(* Logix 5000 AddOnInstructionDefinition export YAI_Assy_72_73_22_23_EIP_Hz; software revision 17.00 *)

ADD_ON_INSTRUCTION YAI_Assy_72_73_22_23_EIP_Hz   (* revision 1.0, vendor Yaskawa America, Inc. *)
// YAI Assembly 72/73 and 22/23
// Speed is given in Hz
// Torque is given in % rated torque
// Help:
// This add-on instruction is for use with input assemblie 72 or 73 and output assemblies 22 or 23.
// Node_Input_Assy is defined as the node's input assembly integer array.
// Node_Output_Assy is defined as the node's output assembly integer array.
// Torque limit/reference and torque output variables are only available with A1000.
VAR_IN_OUT
   Node_Input_Assy : AB:ETHERNET_MODULE_INT_6Bytes:I:0; {required}   // Input assembly words
   Node_Output_Assy : AB:ETHERNET_MODULE_INT_6Bytes:O:0; {required}   // Output assembly words
END_VAR
VAR_INPUT
   RunFwd : BOOL; {visible}   // Forward run command
   RunRev : BOOL; {visible}   // Reverse run command
   FaultReset : BOOL; {visible}   // Fault reset command
   Net_Control : BOOL;   // Network control bit to switch between b1-02 setting and network.
   Net_Ref : BOOL;   // Network reference bit to switch between b1-01 setting and network.
   Freq_Ref : REAL; {visible}   // Frequency reference command in Hz (xx.xx resolution)
   Torq_Ref_Limit : REAL; {visible}   // Torque reference/limit (A1000 only) Engineering Units
END_VAR
VAR_OUTPUT
   Faulted : BOOL; {visible}   // Drive faulted status bit
   Warning : BOOL; {visible}   // Drive warning (alarm) status bit
   RunningFwd : BOOL; {visible}   // Drive running forward status bit
   RunningRev : BOOL; {visible}   // Drive running reverse status bit
   Ready : BOOL; {visible}   // Drive ready status bit
   NetRefStatus : BOOL; {visible}   // Drive network reference status bit (1 = reference coming from network)
   NetCtrlStatus : BOOL; {visible}   // Drive network run source status bit (1 = source coming from network)
   Drive_State : INT;   // Drive Status - Refer to class 0x29, Instance 0x1, Attribute 0x6 for details
   At_Speed : BOOL; {visible}   // Drive at commanded speed status bit
   Output_Freq : REAL; {visible}   // Drive output frequency in Hz (xx.xx resolution)
   Torque_Actual : REAL; {visible}   // Drive torque output in engineering units.
END_VAR
VAR_INPUT
   Motor_Rated_Torq : REAL := 100.0; {visible}   // Motor rated torque (Engineering units)
END_VAR
VAR
   FRef_Convert : DINT;
   FOut_Convert : REAL;
   FOut_Temp : REAL;
   TRef_Convert : INT;
   DriveStatusTempBits : INT;
   TOut_Convert : REAL;
   TOut_Temp : REAL;
   Motor_Torq_Temp : REAL;
   Tout_Convert_Temp : REAL;
END_VAR

ROUTINE Logic   (* ladder *)
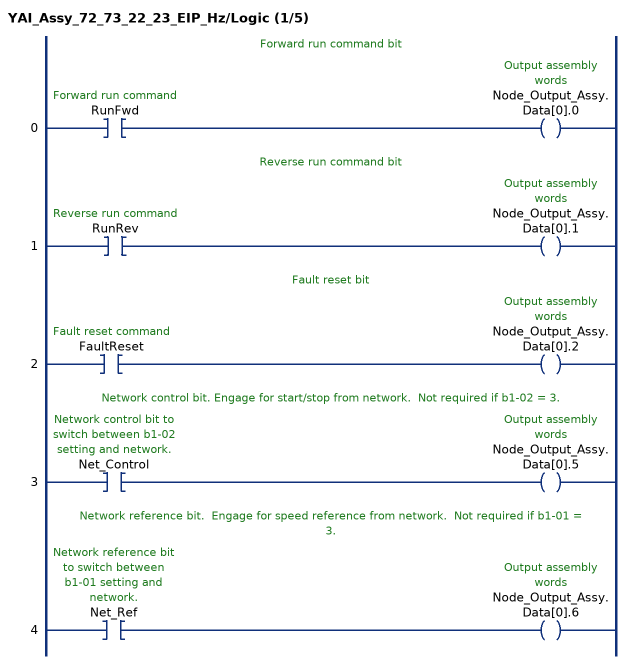
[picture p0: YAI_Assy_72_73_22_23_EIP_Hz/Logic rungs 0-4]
   // Forward run command bit
   0: XIC(RunFwd)OTE(Node_Output_Assy.Data[0].0);
   // Reverse run command bit
   1: XIC(RunRev)OTE(Node_Output_Assy.Data[0].1);
   // Fault reset bit
   2: XIC(FaultReset)OTE(Node_Output_Assy.Data[0].2);
   // Network control bit. Engage for start/stop from network.  Not required if b1-02 = 3.
   3: XIC(Net_Control)OTE(Node_Output_Assy.Data[0].5);
   // Network reference bit.  Engage for speed reference from network.  Not required if b1-01 = 3.
   4: XIC(Net_Ref)OTE(Node_Output_Assy.Data[0].6);
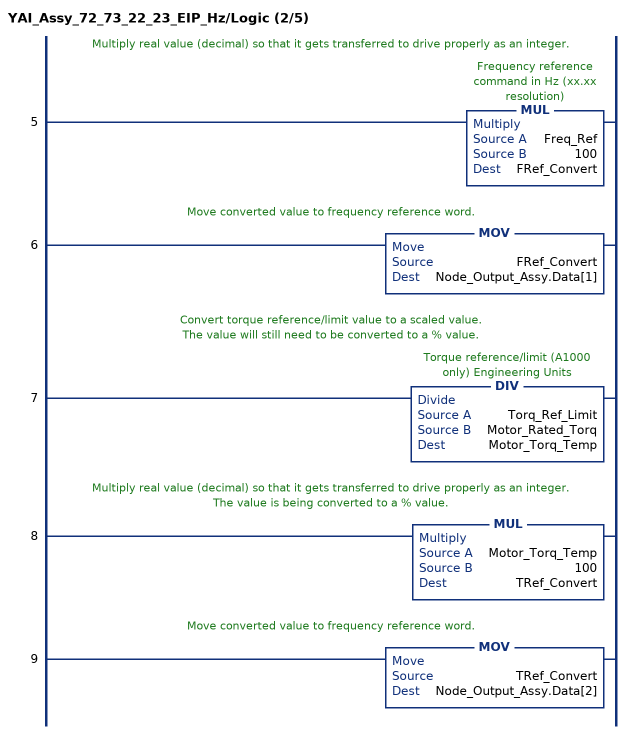
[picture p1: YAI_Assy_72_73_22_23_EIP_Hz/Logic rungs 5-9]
   // Multiply real value (decimal) so that it gets transferred to drive properly as an integer.
   5: MUL(Freq_Ref,100,FRef_Convert);
   // Move converted value to frequency reference word.
   6: MOV(FRef_Convert,Node_Output_Assy.Data[1]);
   // Convert torque reference/limit value to a scaled value.
   // The value will still need to be converted to a % value.
   7: DIV(Torq_Ref_Limit,Motor_Rated_Torq,Motor_Torq_Temp);
   // Multiply real value (decimal) so that it gets transferred to drive properly as an integer.
   // The value is being converted to a % value.
   8: MUL(Motor_Torq_Temp,100,TRef_Convert);
   // Move converted value to frequency reference word.
   9: MOV(TRef_Convert,Node_Output_Assy.Data[2]);
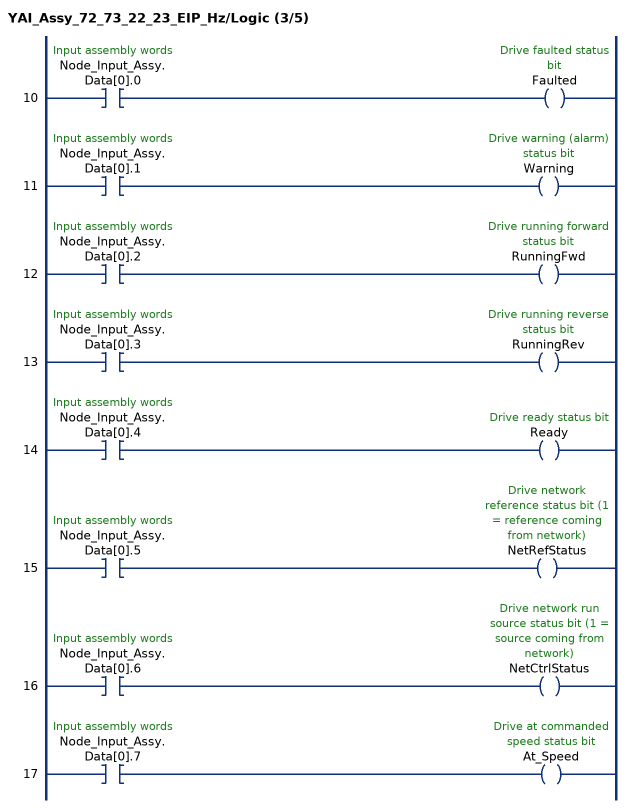
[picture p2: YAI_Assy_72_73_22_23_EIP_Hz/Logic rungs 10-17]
   10: XIC(Node_Input_Assy.Data[0].0)OTE(Faulted);
   11: XIC(Node_Input_Assy.Data[0].1)OTE(Warning);
   12: XIC(Node_Input_Assy.Data[0].2)OTE(RunningFwd);
   13: XIC(Node_Input_Assy.Data[0].3)OTE(RunningRev);
   14: XIC(Node_Input_Assy.Data[0].4)OTE(Ready);
   15: XIC(Node_Input_Assy.Data[0].5)OTE(NetRefStatus);
   16: XIC(Node_Input_Assy.Data[0].6)OTE(NetCtrlStatus);
   17: XIC(Node_Input_Assy.Data[0].7)OTE(At_Speed);
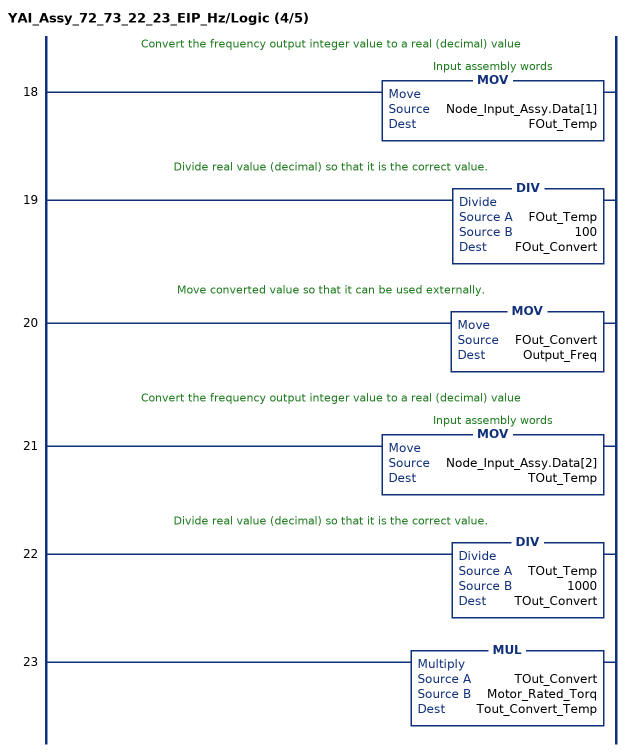
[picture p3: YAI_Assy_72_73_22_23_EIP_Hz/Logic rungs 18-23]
   // Convert the frequency output integer value to a real (decimal) value
   18: MOV(Node_Input_Assy.Data[1],FOut_Temp);
   // Divide real value (decimal) so that it is the correct value.
   19: DIV(FOut_Temp,100,FOut_Convert);
   // Move converted value so that it can be used externally.
   20: MOV(FOut_Convert,Output_Freq);
   // Convert the frequency output integer value to a real (decimal) value
   21: MOV(Node_Input_Assy.Data[2],TOut_Temp);
   // Divide real value (decimal) so that it is the correct value.
   22: DIV(TOut_Temp,1000,TOut_Convert);
   23: MUL(TOut_Convert,Motor_Rated_Torq,Tout_Convert_Temp);
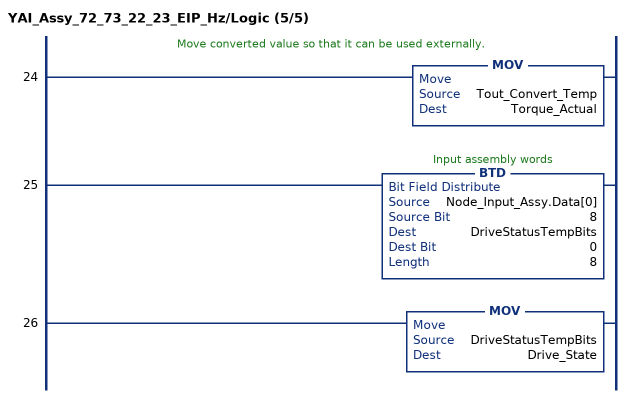
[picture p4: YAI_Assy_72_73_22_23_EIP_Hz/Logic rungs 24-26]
   // Move converted value so that it can be used externally.
   24: MOV(Tout_Convert_Temp,Torque_Actual);
   25: BTD(Node_Input_Assy.Data[0],8,DriveStatusTempBits,0,8);
   26: MOV(DriveStatusTempBits,Drive_State);
END_ROUTINE
END_ADD_ON_INSTRUCTION
